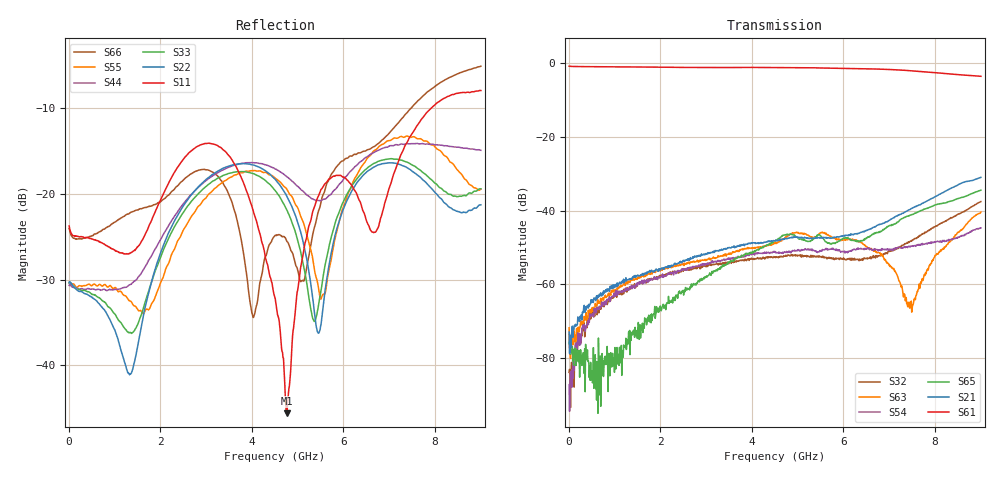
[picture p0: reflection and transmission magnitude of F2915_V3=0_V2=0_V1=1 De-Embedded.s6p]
! Integrated Device Technology
! Corporate Headquarters
! 6024 Silver Creek Valley Road
! San Jose, CA 95138  USA
! Phone:  1-408-284-8200
! Toll Free:  1-800-223-1366
! Webpage:  http://www.idt.com/
! Timing and RF Division
! 515 Groton Road, Suite 102
! Westford, MA 01886-6024
! Device:  F2915
! Description: High Reliability SP5T RF Switch
! Frequency:  0.05 -  8.GHz
! Package:  4x4 mm Thin QFN Plastic Package: 24 pin
! Ports:  6 RF,  5 DC
!  Pin  1  = GND
!  Pin  2  = RF5  =  Port 5
!  Pin  3  = GND
!  Pin  4  = GND
!  Pin  5  = RF4  =  Port 4
!  Pin  6  = GND
!  Pin  7  = GND
!  Pin  8  = RF3  =  Port 3
!  Pin  9  = GND
!  Pin 10  = GND
!  Pin 11  = RF2  =  Port 2
!  Pin 12  = GND
!  Pin 13  = GND
!  Pin 14  = RF1  =  Port 1
!  Pin 15  = GND
!  Pin 16  = Vcc
!  Pin 17  = V1
!  Pin 18  = V2
!  Pin 19  = V3
!  Pin 20  = VSSext
!  Pin 21  = GND
!  Pin 22  = RFC  =  Port 6
!  Pin 23  = GND
!  Pin 24  = GND
! Voltage:  VDD  =  +3.30 Volts
!  VSSEXT =  0.00 Volts
! Current:  IDD  = 252  uA
! State:  RF1 Selected
! V1:  Logic HIGH
! V2:  Logic LOW
! V3:  Logic LOW
! Data:  The device was measured on the F291x evaluation board which has
!  individual transmission lines to the RF pins.  Data was collected
!  using a calibrated network analyzer.  The input lines were
!  modeled using Automatic Fixture Removal (AFR) from Keysight.
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# Hz S  dB  R 50
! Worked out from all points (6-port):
!   900 points, 10 MHz to 9 GHz, reference 50 ohm
!   strongest paths, dB at 10 MHz, 2.26 GHz, 4.51 GHz, 6.76 GHz, 9 GHz:
!     S61: -0.8, -1.1, -1.1, -1.6, -3.5
!     S21: -73.0, -54.9, -48.2, -43.8, -31.0
!     S65: -75.7, -64.2, -48.2, -45.9, -34.4
!     S54: -87.3, -57.0, -51.4, -50.9, -44.7
!     S63: -71.8, -55.1, -48.9, -51.4, -40.4
!     S32: -83.9, -56.8, -52.6, -52.2, -37.5
!   lowest |S11| = -45.6 dB at 4.76 GHz (marker M1), VSWR 1.01, Z = 50.5 - j0.173 ohm
!   |S11| at or under -10 dB: start of sweep to 7.921 GHz
